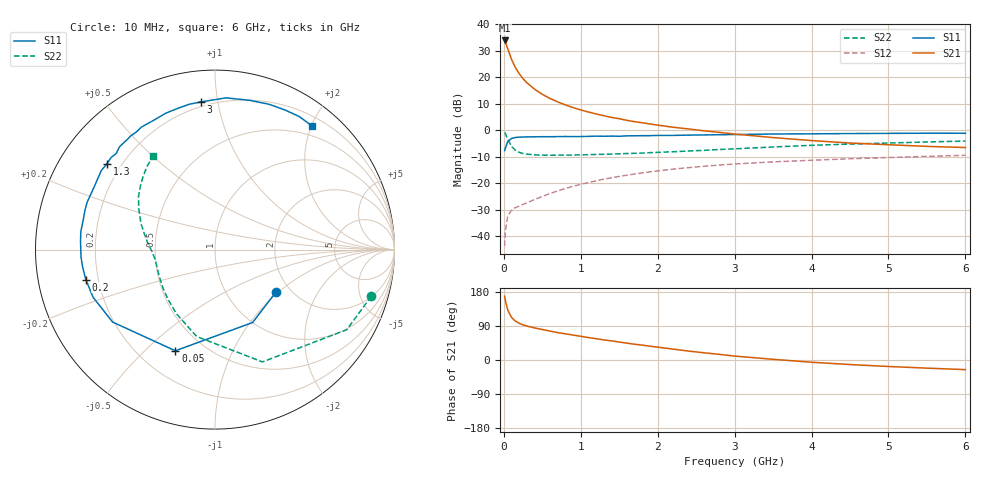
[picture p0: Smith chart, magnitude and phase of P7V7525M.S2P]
! SIEMENS Small Signal Semiconductors
! BFP196
! Si NPN RF Bipolar Junction Transistor in SOT143
! VCE = 0.75 V  IC = 25 mA
! Common Emitter S-Parameters:  May  1996
# GHz  S  MA  R  50
!  f  S11  S21  S12  S22
! GHz  MAG  ANG  MAG  ANG  MAG  ANG  MAG  ANG
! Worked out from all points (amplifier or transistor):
!   36 points, 10 MHz to 6 GHz, reference 50 ohm
!   highest |S21| = 33.8 dB at 10 MHz (marker M1)
!   |S21| within 3 dB of that: start of sweep to 49.27 MHz
!   unconditionally stable (mu >= 1): 545.8 MHz to end of sweep
!   at 250 MHz: K = 0.70, MSG = 23.7 dB, |S12| = -28.0 dB
!   at 1.4 GHz: K = 1.12, MAG = 9.3 dB, |S12| = -18.0 dB
!   at 6 GHz: K = 1.02, MAG = 0.6 dB, |S12| = -9.5 dB
!   S11 on the Smith chart (normalised r, x): 10 MHz: 1.69, -0.96; 50 MHz: 0.35, -0.62; 200 MHz: 0.15, -0.11; 1.3 GHz: 0.15, +0.34; 3 GHz: 0.17, +0.89; 6 GHz: 0.34, +2.00
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0.01  0.414 -34.6  49.22 168.4  0.0065 78.0  0.909 -16.6
0.02  0.4571 -62.7  45.75 156.4  0.0125 69.6  0.8592 -31.3
0.05  0.6055 -111.4  34.6 132.1  0.024 50.0  0.6792 -67.1
0.1  0.6989 -144.7  21.61 112.3  0.031 39.0  0.4947 -101.9
0.15  0.7292 -158.6  15.18 102.7  0.0347 37.8  0.4174 -120.9
0.2  0.7389 -166.9  11.64 96.8  0.0369 39.3  0.382 -133.1
0.25  0.7438 -172.4  9.328 92.7  0.0398 41.0  0.3629 -141.9
0.3  0.7475 -176.6  7.823 89.6  0.0429 43.3  0.3538 -147.5
0.4  0.7506 176.6  5.927 84.6  0.0493 47.1  0.3428 -155.9
0.5  0.7544 172.3  4.746 80.5  0.0565 50.2  0.3384 -161.2
0.6  0.7525 167.5  3.965 76.3  0.0639 51.7  0.3369 -164.8
0.7  0.757 163.1  3.416 72.2  0.0716 52.8  0.338 -167.7
0.9  0.7575 155.6  2.665 65.8  0.0877 53.5  0.34 -172.3
1.1  0.7644 148.4  2.2 59.2  0.1031 52.9  0.3458 -175.4
1.3  0.7684 141.6  1.875 53.0  0.1195 51.6  0.3511 -178.3
1.7  0.7839 129.1  1.446 41.6  0.1492 47.2  0.367 176.3
2.2  0.7973 115.4  1.137 28.8  0.1845 40.7  0.392 170.1
3  0.8265 95.6  0.846 10.4  0.2306 29.4  0.4453 158.7
3.5  0.8477 85.8  0.725 1.8  0.2525 22.8  0.4821 151.8
4.5  0.8639 69.6  0.573 -12.0  0.2888 11.0  0.547 139.4
5.5  0.8773 57.6  0.495 -21.5  0.321 0.5  0.5996 129.0
6  0.8758 52.0  0.471 -25.4  0.336 -5.3  0.6238 123.7
